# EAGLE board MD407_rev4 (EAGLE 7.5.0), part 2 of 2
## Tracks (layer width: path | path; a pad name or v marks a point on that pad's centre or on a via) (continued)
PC4  (via drill 0.4) (continued)
  Top 0.254: v104.5,44.88 105.06,44.88 106.83,43.11 U1.33 111,38.96 111,30 106.6,25.6 106.6,23.5 | v70.25,41 69.12,41 67.5,42.62 RN6.3
  Bottom 0.254: v104.5,44.88 72.75,44.88 71,43.12 71,41.75 v70.25,41
PC5  (via drill 0.4)
  Top 0.2: U3.10 107,23.5
  Top 0.254: v104.5,46.12 107.2,43.43 U1.34 111.5,39.17 111.5,29.75 107,25.25 107,23.5 | v70.25,42.25 69.75,42.75 68.25,42.75 67.58,43.42 RN6.4
  Bottom 0.254: v104.5,46.12 100.62,46.12 99.88,45.38 72.12,45.38 70.25,43.5 v70.25,42.25
PC6
  Top 0.2: U11.8 111.4,77.62
  Top 0.254: U1.63 112.25,59.75 112.25,76 111.4,76.85 111.4,77.62
PC7
  Top 0.2: U11.7 111,77.62
  Top 0.254: U1.64 108.39,56.57 111.75,59.94 111.75,75.75 111,76.5 111,77.62
PC8
  Top 0.2: U11.6 110.6,77.62
  Top 0.254: U1.65 107.99,56.86 111.25,60.12 111.25,75.5 110.6,76.15 110.6,77.62
PC9
  Top 0.2: U11.5 110.2,77.62
  Top 0.254: U1.66 110.75,60.38 110.75,75.25 110.2,75.8 110.2,77.62
PC10  (via drill 0.4)
  Top 0.2: U8.4 102.8,77.62
  Top 0.254: U1.78 98.88,61.7 98.88,64.25 v101.25,66.62 102,67.38 102,74.75 102.8,75.55 102.8,77.62 | v80.12,80.62 79.25,80.62 77.78,79.15 RN4.6
  Bottom 0.254: v101.25,66.62 101.25,68 91.88,77.38 83.38,77.38 v80.12,80.62
PC11  (via drill 0.4)
  Top 0.2: U8.3 102.4,77.62
  Top 0.254: RN4.5 78.58,78.7 79.12,79.25 v80.12,79.25 | U1.79 98.38,61.49 98.38,65 v100,66.62 101.5,68.12 101.5,75 102.4,75.9 102.4,77.62 | v76.38,81.5 74.88,81.5 74.1,80.72 R11.1
  Bottom 0.254: v100,66.62 100,68.5 91.62,76.88 82.5,76.88 v80.12,79.25 77.88,81.5 v76.38,81.5
PC12  (via drill 0.4)
  Top 0.2: U8.2 102,77.62
  Top 0.254: U1.80 97.88,61.28 97.88,66.12 v98.38,66.62 101,69.25 101,75.25 102,76.25 102,77.62 | v77.5,80.25 77.5,80.12 77,79.62 77,78.2 RN4.7
  Bottom 0.254: v98.38,66.62 98.38,69.25 91.25,76.38 81.5,76.38 v77.5,80.25
PC13
  Top 0.2: U2.11 83.6,23.5
  Top 0.254: U1.7 94.38,46.12 93.62,46.12 92.75,45.25 85.5,45.25 83.5,43.25 83.5,25.5 83.6,25.4 83.6,23.5
PC14
  Top 0.2: U2.10 84,23.5
  Top 0.254: U1.8 95.51,46.58 94.56,45.62 93.88,45.62 93,44.75 85.75,44.75 84,43 84,23.5
PC15
  Top 0.2: U2.9 84.4,23.5
  Top 0.254: U1.9 95.87,46.18 94.81,45.12 94.12,45.12 93.25,44.25 86,44.25 84.5,42.75 84.5,25.5 84.4,25.4 84.4,23.5
PD0
  Top 0.2: U8.1 101.6,77.62
  Top 0.254: U1.81 97.38,61.08 97.38,66.88 100.5,70 100.5,75.5 101.6,76.6 101.6,77.62
PD1
  Top 0.2: U10.8 97.4,77.62
  Top 0.254: U1.82 96.88,60.87 96.88,67.12 97.75,68 97.75,69.5 97,70.25 97,73.12 97.4,73.53 97.4,77.62
PD2
  Top 0.2: U10.7 97,77.62
  Top 0.254: U1.83 96.38,60.66 96.38,67.38 97.25,68.25 97.25,69.25 96.5,70 96.5,73.38 97,73.88 97,77.62
PD3  (via drill 0.4)
  Top 0.2: U10.6 96.6,77.62
  Top 0.254: U1.84 95.88,60.45 95.88,68.25 v96.38,68.75 96,69.12 96,73.62 96.6,74.22 96.6,77.62 | v76.12,80.25 76.17,80.2 RN4.8 75.67,78.17 74.75,77.25 R9.1
  Bottom 0.254: v96.38,68.75 89.38,75.88 81.25,75.88 77.62,79.38 77,79.38 v76.12,80.25
PD4
  Top 0.2: U10.5 96.2,77.62
  Top 0.254: U1.85 95.38,60.25 95.38,73.75 96.2,74.58 96.2,77.62
PD5
  Top 0.2: U10.4 95.8,77.62
  Top 0.254: U1.86 94.88,60.04 94.88,74 95.8,74.92 95.8,77.62
PD6
  Top 0.2: U10.3 95.4,77.62
  Top 0.254: U1.87 94.38,59.83 94.38,74.25 95.4,75.28 95.4,77.62
PD7
  Top 0.2: U10.2 95,77.62
  Top 0.254: U1.88 93.88,59.62 93.88,74.5 95,75.62 95,77.62
PD8
  Top 0.2: U9.8 118.4,77.62
  Top 0.254: U1.55 111.58,53.39 116.25,58.06 116.25,72.25 118.4,74.4 118.4,77.62
PD9
  Top 0.2: U9.7 118,77.62
  Top 0.254: U1.56 111.18,53.74 115.75,58.31 115.75,72.5 118,74.75 118,77.62
PD10
  Top 0.2: U9.6 117.6,77.62
  Top 0.254: U1.57 115.25,58.5 115.25,72.75 117.6,75.1 117.6,77.62
PD11
  Top 0.2: U9.5 117.2,77.62
  Top 0.254: U1.58 110.42,54.42 114.75,58.75 114.75,73 117.2,75.45 117.2,77.62
PD12
  Top 0.2: U9.4 116.8,77.62
  Top 0.254: U1.59 110.12,54.74 114.25,58.88 114.25,73.25 116.8,75.8 116.8,77.62
PD13
  Top 0.2: U9.3 116.4,77.62
  Top 0.254: U1.60 113.75,59.12 113.75,73.5 116.4,76.15 116.4,77.62
PD14
  Top 0.2: U9.2 116,77.62
  Top 0.254: U1.61 109.36,55.49 113.25,59.38 113.25,73.75 116,76.5 116,77.62
PD15
  Top 0.2: U9.1 115.6,77.62
  Top 0.254: U1.62 108.99,55.8 112.69,59.5 112.75,74 115.6,76.85 115.6,77.62
PE0
  Top 0.2: U7.2 88,77.62
  Top 0.254: U1.97 92.89,54.25 91.25,54.25 89.88,55.62 89.88,72.88 88.38,74.38 88.25,74.5 88,74.75 88,77.62
PE1
  Top 0.2: U7.1 87.6,77.62
  Top 0.254: U1.98 92.68,53.75 91,53.75 89.38,55.38 89.38,72.62 87.6,74.4 87.6,77.62
PE2
  Top 0.2: U2.16 81.6,23.5
  Top 0.254: U1.1 93.09,49.09 91.75,47.75 84.25,47.75 81,44.5 81,24.38 81.6,23.77 81.6,23.5
PE3
  Top 0.2: U2.15 82,23.5
  Top 0.254: U1.2 93.45,48.7 92,47.25 84.5,47.25 81.5,44.25 81.5,24.62 82,24.12 82,23.5
PE4
  Top 0.2: U2.14 82.4,23.5
  Top 0.254: U1.3 93.75,48.31 92.19,46.75 84.75,46.75 82,44 82,24.88 82.4,24.48 82.4,23.5
PE5
  Top 0.2: U2.13 82.8,23.5
  Top 0.254: U1.4 92.38,46.25 85,46.25 82.5,43.75 82.5,25.12 82.8,24.82 82.8,23.5
PE6
  Top 0.2: U2.12 83.2,23.5
  Top 0.254: U1.5 94.48,47.67 92.56,45.75 85.25,45.75 83,43.5 83,25.38 83.2,25.18 83.2,23.5
PE7
  Top 0.2: U5.14 112.4,23.5
  Top 0.254: U1.38 113.5,40 113.5,26.88 112.4,25.77 112.4,23.5
PE8
  Top 0.2: U5.13 112.8,23.5
  Top 0.254: U1.39 114,40.21 114,26.62 112.8,25.43 112.8,23.5
PE9
  Top 0.2: U5.12 113.2,23.5
  Top 0.254: U1.40 114.5,40.41 114.5,26.38 113.2,25.07 113.2,23.5
PE10
  Top 0.2: U5.11 113.6,23.5
  Top 0.254: U1.41 115,40.62 115,26.12 113.6,24.73 113.6,23.5
PE11
  Top 0.2: U5.10 114,23.5
  Top 0.254: U1.42 115.5,40.83 115.5,25.88 114,24.38 114,23.5
PE12
  Top 0.2: U5.9 114.4,23.5
  Top 0.254: U1.43 116,41.04 116,25.62 114.4,24.02 114.4,23.5
PE13
  Top 0.2: U4.16 118.6,23.5
  Top 0.254: U1.44 116.5,41.24 116.5,26.88 118.6,24.77 118.6,23.5
PE14
  Top 0.2: U4.15 119,23.5
  Top 0.254: U1.45 117,41.45 117,27.12 119,25.12 119,23.5
PE15
  Top 0.2: U4.14 119.4,23.5
  Top 0.254: U1.46 117.5,41.66 117.5,27.38 119.4,25.48 119.4,23.5
SW  (via drill 0.4)
  Top 0.254: C40.2 v24.38,89.5 | U21.10 28.61,84.61 28.62,84.62 28.75,84.62 29,84.88 29,86 29.12,86.12 | D2.C 31.18,86.08 32.88,84.38 L1.1 | L1.1 34.62,84.5 | v34.62,86.12 L1.1
  Bottom 0.254: v24.38,89.5 30.5,89.5 32.12,87.88 33.12,87.88 34.62,86.38 v34.62,86.12
  pour Top (isolate 0.305): 27.75,84 27.75,87.75 35.75,87.75 35.75,83 31.62,83 31.62,83.88 31.62,84
SW_OUT
  Top 0.254: R34.2 38.14,82.77 39,83.62 39,91 | R33.1 44.23,90.72 43.5,90 F1.2
  pour Top (isolate 0.3): 31.12,94.38 31.12,89 44.25,89 44.25,94.38
USB_PWR  (via drill 0.4)
  Top 0.254: v21.91,60.96 21.59,60.64 21.59,59.14 U18.12 21.59,59.12 21.59,57.28 22.25,56.62 22.25,55 23.25,54 23.87,54 23.88,53.99 33.8,53.99 34.02,54.21 R25.2 R26.2 | C31.2 17.12,57.77 v18.41,59.05
  Top 1.016: R16.2 v16.25,70.12 | v41.38,73.12 41.38,75.5 F2.2
  Bottom 0.254: v21.91,60.96 21.59,60.64 20,60.64 v18.41,59.05 18.41,69.46 17.75,70.12 v16.25,70.12
  Bottom 1.016: v16.25,70.12 16.25,72 17.38,73.12 v41.38,73.12
X_NRST
  Top 0.2: X1.11 84.89,8.73 84,9.62 84,11.88 90,17.88 91.75,17.88 93.6,19.73 U6.1
X_PA0
  Top 0.2: X1.16 90.3,13.93 91.62,15.25 92.25,15.25 95.6,18.6 U6.6
X_PA1
  Top 0.2: X1.17 92.64,8.73 91.62,9.75 91.62,14 96,18.38 U6.7
X_PA2
  Top 0.2: X1.18 92.84,14.59 96.4,18.15 U6.8
X_PA3
  Top 0.2: X1.19 95.14,8.73 94.12,9.75 94.12,13.5 99.75,19.12 102.88,19.12 104.6,20.85 U3.1
X_PA4
  Top 0.2: X1.20 95.38,14.01 100,18.62 103,18.62 105,20.62 U3.2
X_PA5
  Top 0.2: X1.21 97.89,8.73 96.62,10 96.62,14.62 100.12,18.12 103.12,18.12 105.4,20.4 U3.3
X_PA6
  Top 0.2: X1.22 97.92,15.29 100.25,17.62 103.25,17.62 105.8,20.18 U3.4
X_PA7
  Top 0.2: X1.23 100.39,8.73 99.12,10 99.12,14.5 101.75,17.12 103.38,17.12 106.2,19.95 U3.5
X_PA8
  Top 0.2: X6.31 110.62,82.12 109.8,81.3 U11.13
X_PA9
  Top 0.2: X6.32 110.62,90.62 109.38,89.38 109.38,79.65 U11.14
X_PA10
  Top 0.2: U11.15 109,86.25 108.12,87.12 108.12,88.69 X6.29
X_PA11
  Top 0.2: X6.30 108.08,90.83 106.88,89.62 106.88,87.75 108.62,86 108.62,79.65 U11.16
X_PA12
  Top 0.2: X6.27 105.54,81.29 104.4,80.15 U8.9
X_PA13
  Top 0.2: X6.28 105.54,90.54 104.25,89.25 104.25,80.62 104,80.38 U8.10
X_PA14
  Top 0.2: X6.25 103,88.12 103.6,87.53 U8.11
X_PA15
  Top 0.2: X6.26 103,90.88 101.75,89.62 101.75,88.25 103.2,86.8 U8.12
X_PB0
  Top 0.2: X1.26 103,14.88 107.4,19.27 U3.8
X_PB1
  Top 0.2: X1.27 104.38,9.89 104.38,13.75 108.88,18.25 110.12,18.25 111.6,19.73 U5.1
X_PB2
  Top 0.2: X1.28 105.54,14.29 109.12,17.88 110.38,17.88 112,19.5 U5.2
X_PB3
  Top 0.2: U10.16 94.6,80.9 88.12,87.38 87.12,87.38 86.5,88 86.5,90.01 X6.14
X_PB4
  Top 0.2: X6.11 85.22,87.66 86.38,86.5 88.25,86.5 90.4,84.35 U7.9
X_PB5
  Top 0.2: U7.10 90,84.12 88.12,86 85.88,86 84,87.88 84,90.05 X6.12
X_PB6
  Top 0.2: U7.11 89.6,83.9 88,85.5 84.88,85.5 82.68,87.69 X6.9
X_PB7
  Top 0.2: U7.12 89.2,83.67 87.88,85 84.5,85 81.5,88 81.5,90.09 X6.10
X_PB8
  Top 0.2: U7.13 88.8,83.45 87.75,84.5 83.25,84.5 80.12,87.62 80.12,88.72 X6.7
X_PB9
  Top 0.2: U7.14 88.4,83.22 87.62,84 82.5,84 78.88,87.62 78.88,90 X6.8
X_PB10
  Top 0.2: U4.4 119.8,19.05 118.25,17.5 X1.38
X_PB11
  Top 0.2: U4.5 120.2,18.82 119.5,18.12 119.5,10.01 X1.39
X_PB12
  Top 0.2: X6.47 130.94,83.69 129.38,82.12 125.62,82.12 123.8,80.3 U12.13
X_PB13
  Top 0.2: X6.48 130.94,90.56 129.75,89.38 129.75,83 129.25,82.5 125.38,82.5 123.4,80.53 U12.14
X_PB14
  Top 0.2: X6.45 128.4,83.65 127.62,82.88 125.12,82.88 123,80.75 U12.15
X_PB15
  Top 0.2: X6.46 128.4,90.4 127.12,89.12 127.12,83.88 126.5,83.25 125,83.25 122.6,80.85 U12.16
X_PC0  (via drill 0.4)
  Top 0.2: X1.12 85.22,12.1 90.5,17.38 91.88,17.38 94,19.5 U6.2
  Top 0.254: v86.62,25.88 v86.62,17.75
  Bottom 0.254: JP1.2 61.66,24.79 62.75,25.88 v86.62,25.88 | v86.62,17.75 85.25,16.38 85.25,11.3 X1.12
X_PC1
  Top 0.2: X1.13 87.52,8.73 86.5,9.75 86.5,12.62 90.75,16.88 92,16.88 94.4,19.27 U6.3
X_PC2  (via drill 0.4)
  Top 0.2: X1.14 87.76,13.13 91,16.38 92.12,16.38 94.8,19.05 U6.4
  Top 0.254: v87.38,24.88 87.38,17.38 v86.62,16.62
  Bottom 0.254: JP1.4 61.25,22.25 62.12,23.12 62.12,24.5 63,25.38 85.75,25.38 86.25,24.88 v87.38,24.88 | v86.62,16.62 85.75,15.75 85.75,13.25 85.88,13.12 86.62,12.4 X1.14
X_PC3  (via drill 0.4)
  Top 0.2: X1.15 90.14,8.73 89,9.88 89,13.62 91.12,15.75 92.12,15.75 95.2,18.82 U6.5
  Top 0.254: v88.12,24.12 88.12,17 v86.62,15.5
  Bottom 0.254: JP1.6 61.46,19.71 62.62,20.88 62.62,24.25 63.25,24.88 85.5,24.88 86.25,24.12 v88.12,24.12 | v86.62,15.5 86.62,14.62 89,12.25 89,10.03 X1.15
X_PC4
  Top 0.2: X1.24 100.46,15.21 101.88,16.62 103.5,16.62 106.6,19.73 U3.6
X_PC5
  Top 0.2: X1.25 102.77,8.73 101.75,9.75 101.75,14.25 107,19.5 U3.7
X_PC6
  Top 0.2: X6.35 115.7,84.7 111.4,80.4 U11.9
X_PC7
  Top 0.2: X6.36 115.7,90.7 114.5,89.5 114.5,84.12 111,80.62 U11.10
X_PC8
  Top 0.2: X6.33 113.16,83.41 110.6,80.85 U11.11
X_PC9
  Top 0.2: X6.34 113.16,90.66 111.88,89.38 111.88,82.75 110.2,81.08 U11.12
X_PC10
  Top 0.2: X6.23 100.52,88.73 102.8,86.45 U8.13
X_PC11
  Top 0.2: X6.24 100.46,90.58 99.25,89.38 99.25,87.38 102,84.62 102.38,84.25 102.4,84.22 U8.14
X_PC12
  Top 0.2: X6.21 97.92,88.08 102,84 U8.15
X_PC13
  Top 0.2: U2.6 83.6,17.23 80.14,13.77 X1.8
X_PC14
  Top 0.2: U2.7 84,16.75 81.5,14.25 81.5,9.91 X1.9
X_PC15
  Top 0.2: U2.8 84.4,16.15 82.68,14.43 X1.10
X_PD0  (via drill 0.4)
  Top 0.2: U8.16 101.6,83.4 96.75,88.25 96.75,90.1 X6.22
  Top 0.254: X4.2 138.04,78.42 v138,78
  Bottom 0.254: X6.22 96.75,90.1 96.75,88.12 98.88,86 134.62,86 v136.5,87.88 138,86.38 v138,78
X_PD1  (via drill 0.4)
  Top 0.2: U10.9 97.4,86.22 95.44,88.19 95.44,88.67 X6.19
  Top 0.254: v143.38,86.12 143,86.5 v136.5,86.5
  Bottom 0.254: X6.19 95.38,88.25 98.25,85.38 134.75,85.38 135.88,86.5 v136.5,86.5 | X4.3 153.98,82.25 152.12,82.25 151.5,81.62 151.5,80.75 150.38,79.62 147,79.62 144.38,82.25 144.38,85.12 v143.38,86.12
X_PD2  (via drill 0.4)
  Top 0.2: U10.10 97,85 94.12,87.88 94.12,90.02 X6.20
  Top 0.254: v143.38,84.62 142.88,85.12 v136.5,85.12
  Bottom 0.254: v136.5,85.12 135.25,85.12 135,84.88 97.12,84.88 94.12,87.88 94.12,90.02 X6.20 | v143.38,84.62 143.38,82.5 146.75,79.12 151.38,79.12 152.73,80.48 X4.4
X_PD3  (via drill 0.4)
  Top 0.2: U10.11 96.6,84.03 92.88,87.75 92.88,88.69 X6.17
  Top 0.254: v145.25,84.38 144.62,83.75 v136.5,83.75
  Bottom 0.254: v136.5,83.75 135.5,83.75 134.88,84.38 96.88,84.38 93.31,87.94 93.31,88.26 X6.17 | X4.5 154.15,84.62 151.88,84.62 150.38,83.12 150.38,81.38 149.75,80.75 147.62,80.75 146.12,82.25 146.12,84 145.75,84.38 v145.25,84.38
X_PD4  (via drill 0.4)
  Top 0.2: U10.12 96.2,83.67 91.75,88.12 91.75,90.18 X6.18
  Top 0.254: v145.25,82.88 144.75,82.38 v136.5,82.38
  Bottom 0.254: v136.5,82.38 136,82.38 134.5,83.88 96,83.88 91.62,88.25 91.62,90.06 X6.18 | X4.6 151.75,83.5 151,82.88 151,81.12 150,80.12 147.38,80.12 145.25,82.25 v145.25,82.88
X_PD5  (via drill 0.4)
  Top 0.2: U10.13 95.8,83.23 X6.15
  Top 0.254: v136.5,80.88 147.5,80.88 148.25,81.62 148.25,83 v149.12,83.88
  Bottom 0.254: v136.5,80.88 136.5,81 134.12,83.38 95.38,83.38 90.5,88.25 90.5,88.53 X6.15 | X4.7 154.12,87.25 152.12,87.25 151.25,86.38 151.25,86 v149.12,83.88
X_PD6  (via drill 0.4)
  Top 0.2: U10.14 95.4,81.6 89.12,87.88 89.12,90.09 X6.16
  Top 0.254: v136.5,79.38 137.38,80.25 148.5,80.25 149.12,80.88 v149.12,81.62
  Bottom 0.254: v136.5,79.38 136.5,79.5 133.12,82.88 94,82.88 89.12,87.75 89.12,90.09 X6.16 | v149.12,81.62 149.5,81.62 149.88,82 149.88,83.5 152.41,86.04 X4.8
X_PD7  (via drill 0.4)
  Top 0.2: U10.15 95,81.12 88.25,87.88 88.25,88.24 X6.13
  Top 0.254: v136.5,77.88 138.25,79.62 148.88,79.62 150.38,81.12 150.38,82.38 150,82.75 v149.12,82.75
  Bottom 0.254: v136.5,77.88 136.38,77.88 131.88,82.38 93.75,82.38 87.94,88.19 87.94,88.55 X6.13 | X4.9 154.06,89.75 151,89.75 148.12,86.88 148.12,83.12 148.5,82.75 v149.12,82.75
X_PD8
  Top 0.2: X6.43 125.86,84.11 125.38,83.62 121.75,83.62 118.4,80.28 U9.9
  Bottom 0.254: X6.43 127.12,90 127.12,92 127.62,92.5 134.25,92.5 139,87.75 139,76.5 147.12,68.38 147.12,58.62 149.33,56.42 X3.2
X_PD9
  Top 0.2: X6.44 125.86,90.86 124.62,89.62 124.62,85.25 123.38,84 121.5,84 118,80.5 U9.10
  Bottom 0.254: X6.44 125.86,92.11 126.75,93 134.5,93 139.5,88 139.5,76.75 147.62,68.62 147.62,59.38 149.25,57.75 154.06,57.75 X3.3
X_PD10
  Top 0.2: X6.41 123.32,84.82 122.88,84.38 121.25,84.38 117.6,80.72 U9.11
  Bottom 0.254: X6.41 124.62,90.03 124.62,92.38 125.75,93.5 134.75,93.5 140,88.25 140,77 148.12,68.88 148.12,60.25 149.41,58.96 X3.4
X_PD11
  Top 0.2: X6.42 123.32,90.69 122,89.38 122,85.25 121.5,84.75 121,84.75 117.2,80.95 U9.12
  Bottom 0.254: X6.42 123.32,92.44 124.88,94 135,94 140.5,88.5 140.5,77.25 148.62,69.12 148.62,61.5 149.88,60.25 154.02,60.25 X3.5
X_PD12
  Top 0.2: X6.39 120.78,85.16 116.8,81.17 U9.13
  Bottom 0.254: X6.39 122,89.95 122,92.5 124,94.5 135.25,94.5 141,88.75 141,77.5 149.12,69.38 149.12,62.5 150.12,61.5 X3.6
X_PD13
  Top 0.2: X6.40 120.78,90.66 119.5,89.38 119.5,84.5 116.4,81.4 U9.14
  Bottom 0.254: X6.40 120.78,92.66 123.12,95 135.5,95 141.5,89 141.5,77.75 149.62,69.62 149.62,64 150.88,62.75 153.98,62.75 X3.7
X_PD14
  Top 0.2: X6.37 118.24,83.86 116,81.62 U9.15
  Bottom 0.254: X6.37 119.5,89.99 119.5,92.62 122.38,95.5 135.75,95.5 142,89.25 142,78 150.12,69.88 150.12,65.12 151.21,64.04 X3.8
X_PD15
  Top 0.2: X6.38 118.24,90.49 117,89.25 117,83.25 115.6,81.85 U9.16
  Bottom 0.254: X6.38 118.24,92.49 121.75,96 136,96 142.5,89.5 142.5,78.25 150.62,70.12 150.62,66.25 151.62,65.25 153.94,65.25 X3.9
X_PE0
  Top 0.2: U7.15 88,82.88 87.38,83.5 81.88,83.5 77.75,87.62 77.75,88.58 X6.5
  Bottom 0.254: X6.5 77.75,88.58 77.75,87.62 84.38,81 118.38,81 121.5,77.88 133.75,77.88 146.5,65.12 146.5,57.5 149.5,54.5 153.88,54.5 155.88,52.5 155.88,47.5 157,46.38 157,37 155.62,35.62 153.88,35.62 152.73,34.48 X5.2
X_PE1
  Top 0.2: U7.16 87.6,82.53 87.12,83 81.5,83 76.38,88.12 76.38,90.05 X6.6
  Bottom 0.254: X6.6 76.38,90.05 76.38,88.12 84.25,80.25 118.38,80.25 121.25,77.38 133.5,77.38 146,64.88 146,57.25 149.25,54 153.62,54 155.38,52.25 155.38,47.25 156.5,46.12 156.5,37.88 155.59,36.96 X5.3
X_PE2  (via drill 0.4)
  Top 0.2: 75.06,9.19 73.88,10.38 73.88,13.5 79.12,18.75 80.38,18.75 81.6,19.98 U2.1
  Top 0.254: X5.4 152.73,36.48 150.5,34.25 v149,34.25 | X1.3 75.06,9.19
  Bottom 0.254: X1.3 75.06,8.06 75.75,7.38 80.75,7.38 81.5,8.12 81.5,15.62 84.38,18.5 139.88,18.5 146.5,25.12 146.5,33.12 147.62,34.25 v149,34.25
X_PE3
  Top 0.2: U2.2 82,19.5 75,12.5 75,11.33 X1.4
  Bottom 0.254: X1.4 75,11.33 75,13.62 75.12,13.75 81.5,20 139.12,20 145,25.88 145,35.12 148.38,38.5 151.5,38.5 151.75,38.25 154.02,38.25 X5.5
X_PE4
  Top 0.2: U2.3 82.4,18.77 76.38,12.75 76.38,9.96 X1.5
  Bottom 0.254: X1.5 76.33,10 74.25,10 73.88,10.38 73.88,13.88 80.62,20.5 138.88,20.5 144.5,26.12 144.5,35.38 148.12,39 152.23,39 X5.6
X_PE5  (via drill 0.4)
  Top 0.2: U2.4 82.8,18.3 77.62,13.12 77.62,11.29 X1.6
  Top 0.254: v149,36.5 150.12,36.5 150.88,37.25 150.88,42.25 151.88,43.25 154.06,43.25 X5.7
  Bottom 0.254: X1.6 77.62,11.29 77.62,14.62 82.75,19.5 139.38,19.5 145.5,25.62 145.5,34.38 147.62,36.5 v149,36.5
X_PE6  (via drill 0.4)
  Top 0.2: U2.5 83.2,17.7 78.88,13.38 78.88,9.99 X1.7
  Top 0.254: v149,35.38 150.38,35.38 151.5,36.5 151.5,40.81 X5.8
  Bottom 0.254: X1.7 78.88,9.99 78.88,14 83.88,19 139.62,19 146,25.38 146,33.75 147.75,35.38 v149,35.38
X_PE7  (via drill 0.4)
  Top 0.2: X1.29 107.89,8.73 106.88,9.75 106.88,15 109.25,17.38 110.5,17.38 112.4,19.27 U5.3
  Top 0.254: v149,37.62 v149,40
  Bottom 0.254: X1.29 106.88,9.94 106.88,14.5 110.38,18 140.12,18 147,24.88 147,32.38 148,33.38 149.38,33.38 150.5,34.5 150.5,36.5 149.38,37.62 v149,37.62 | v149,40 149,40.38 151.88,43.25 153.94,43.25 X5.9
X_PE8
  Top 0.2: X1.30 108.12,11.31 108.12,15.62 109.38,16.88 110.62,16.88 112.8,19.05 U5.4
  Bottom 0.254: X1.30 108.08,12.21 113,17.12 149.88,17.12 151.5,18.75 156.25,18.75 156.62,18.38 156.62,14.12 156.12,13.62 153.94,13.62 X7.2
X_PE9
  Top 0.2: X1.31 109.5,9.85 109.5,15.5 110.5,16.5 110.88,16.5 113.2,18.82 U5.5
  Bottom 0.254: X1.31 111.88,9.98 111.88,12.25 115.75,16.12 149.38,16.12 151.88,13.62 153.12,13.62 154.25,14.75 155.06,14.75 X7.3
X_PE10
  Top 0.2: X1.32 110.62,15.62 113.6,18.6 U5.6
  Bottom 0.254: X1.32 110.62,12.37 114.88,16.62 151.12,16.62 151.5,16.25 151.5,15.75 152.41,14.96 X7.4
X_PE11  (via drill 0.4)
  Top 0.2: U5.7 114,18.38 111.88,16.25 111.88,10.02 X1.33
  Top 0.254: X7.5 155.27,17.61 154.12,18.75 149.62,18.75 147.5,16.62 147.5,14.5 v148.62,13.38
  Bottom 0.254: X1.33 114.38,9.95 114.38,12.38 117.12,15.12 146.88,15.12 v148.62,13.38
X_PE12  (via drill 0.4)
  Top 0.2: U5.8 114.4,18.15 113.12,16.88 113.12,11.3 X1.34
  Top 0.254: X7.6 151.38,17.5 151,17.12 151,15.38 150.38,14.75 v148.62,14.75
  Bottom 0.254: X1.34 113.16,12.79 116,15.62 147.75,15.62 v148.62,14.75
X_PE13  (via drill 0.4)
  Top 0.2: U4.1 118.6,19.73 114.62,15.75 114.62,9.8 X1.35
  Top 0.254: X7.7 155.27,20.23 154.25,21.25 150.25,21.25 146,17 146,12.5 146.62,11.88 v146.88,11.88
  Bottom 0.254: X1.35 117,10.03 117,12 119.12,14.12 144.62,14.12 v146.88,11.88
X_PE14  (via drill 0.4)
  Top 0.2: U4.2 119,19.5 115.62,16.12 115.62,11.35 X1.36
  Top 0.254: X7.8 150.12,20.04 146.88,16.79 146.88,13.12 148,12 v148.62,12
  Bottom 0.254: X1.36 115.7,12.45 117.88,14.62 146,14.62 v148.62,12
X_PE15  (via drill 0.4)
  Top 0.2: U4.3 119.4,19.27 117,16.88 117,9.97 X1.37
  Top 0.254: v147.62,19.75 145.38,17.5 145.38,12.12 v145.12,11.88
  Bottom 0.254: X1.37 119.5,9.99 119.5,11.75 121.38,13.62 143.38,13.62 v145.12,11.88 | X7.9 155.27,22.39 154.12,21.25 149.12,21.25 v147.62,19.75

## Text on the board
tPlace: 5V | GND | PE1 | PB9 | PB7 | PB5 | PB3 | PD6 | PD4 | PD2 | PD0 | PC11 | PA15 | PA13 | PA11 | PA9 | PC9 | PC7 | PD15 | PD13 | PD11 | PD9 | PB15 | PB13 | GND | Overload | B | 3.3V | GND | PE0 | PB8 | PB6 | PB4 | PD7 | PD5 | PD3 | PD1 | PC12 | PC10 | PA14 | PA12 | PA10 | PA8 | PC8 | PC6 | PD14 | PD12 | PD10 | PD8 | PB14 | PB12 | GND | EXT | max 1A | PD0-7 | PWR ON | USB | MAX 50V / DC INPUT | max 0.4A | USB1 | JTAG | PD8-15 | TX | RX | USB2 | User | Reset | MD407 Rev.4 | CHALMERS | 2015-03-28 | PE0-7 | 1 | 2 | CAN1 | CAN2 | 3 | 5V | PE3 | PE5 | PC13 | PC15 | PC0 | PC2 | PA0 | PA2 | PA4 | PA6 | PC4 | PB0 | PB2 | PE8 | PE10 | PE12 | PE14 | PB10 | 3.3V | 3.3V | 3.3V | 3.3V | GND | GND | PE8-15 | A | 3.3V | PE2 | PE4 | PE6 | PC14 | NRST | PC1 | PC3 | PA1 | PA3 | PA5 | PA7 | PC5 | PB1 | PE7 | PE9 | PE11 | PE13 | PE15 | PB11 | 3.3V | 3.3V | 3.3V | GND | GND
